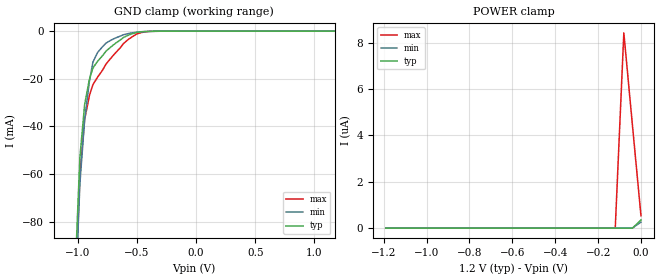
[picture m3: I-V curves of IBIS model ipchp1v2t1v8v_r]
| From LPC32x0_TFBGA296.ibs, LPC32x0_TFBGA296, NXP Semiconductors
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| |   Rev 0.20 IBIS Model Design Automation Generation   |
| |   N O N - S I L I C O N   C O R R E L A T E D   |
| |   This IBIS [Model] is pre-Beta tactical support   |
| |  Note: this IBIS [Model] contains clamp curves generated   |
| |   through simulation which should not be relied upon   |
| ipchp1v2t1v8v
|   Input Pad 1v2
|   Push Pull
|   CMOS
|   Programmable between
|   - (p1=0, p2=1) plain input
|   - (p1=0, p2=0) with Pull Up
|   - (p1=1, p2=1) with Pull Down
|   - (p1=1, p2=0) with Repeater
|   Characterized at Core 1.2V and I/O 1.8V
| Repeater Mode (p1=1, p2=0)
[Model]   ipchp1v2t1v8v_r | of ipchp1v2t1v8v
Model_type   Input
|  Reciever Thresholds
Vinl   = 0.36V
Vinh   = 0.84V
| [Process Range]   typical   min   max
| C_comp edge width   400.000ps   400.000ps   400.000ps
| C_comp Tstrobe   40.000fs   40.000fs   40.000fs
C_comp   2.019pF   1.888pF   2.187pF
[Temperature Range]   25   105   -20
[Voltage Range]   1.20V   1.10V   1.30V
[GND Clamp Reference]   0.00V   0.00V   0.00V
[Pulldown Reference]   0.00V   0.00V   0.00V
[POWER Clamp Reference]   1.20V   1.10V   1.30V
[Pullup Reference]   1.20V   1.10V   1.30V
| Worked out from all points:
|   GND clamp passes 1 mA (typ) near -0.53 V on its own axis
[GND Clamp]
| ref voltage   0.00V   0.00V   0.00V
|   Voltage   I(typ)   I(min)   I(max)
-1.2V     -373.8mA   -377.3mA   -396.4mA
-1.01V    -89.19mA   -101.8mA   -99.48mA
-980mV    -53.07mA   -64.23mA   -60.47mA
-940mV    -30.85mA   -37.28mA   -37.23mA
-900mV    -20.3mA    -21.21mA   -27.11mA
-870mV    -15.47mA   -13mA      -22.46mA
-830mV    -12.6mA    -8.915mA   -19.26mA
-760mV    -8.431mA   -5.043mA   -13.88mA
-570mV    -1.655mA   -988uA     -3.435mA
-500mV    -508.1uA   -391.7uA   -1.156mA
-420mV    -133.8uA   -139.1uA   -246.8uA
1.17V     -2.217uA   4.528nA    -12.6uA
[Power Clamp]   | Vtable = Vcc - Vpad
| ref voltage   1.20V   1.10V   1.30V
|   Voltage   I(typ)   I(min)   I(max)
-1.19V    523.6pA    5.399nA    478.3pA
-120mV    332.3pA    4.574nA    207pA
-80mV     327.9pA    4.541nA    8.428uA
-40mV     323.1pA    4.489nA    4.455uA
0V        354.1nA    261.6nA    531.4nA
